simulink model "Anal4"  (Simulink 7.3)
settings: Solver=ode45  StartTime=0.0  StopTime=10.0  RelTol=1e-3
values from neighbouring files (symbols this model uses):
  d2r = 1/r2d    (= 0.0174532925199)    [run.m]
  Kp3 = [0.3042  3.4539  0.5105  0.0711 -0.2670]    [run.m]
  Thr = [470000, 470000, 470000, 0.245e7, 0.245e7]'    [run.m]
undefined symbols (not defined in the file or in its folder): Ap, Bp, Cp, Cza, Dp, Mass, Qbar, Sref, TVC

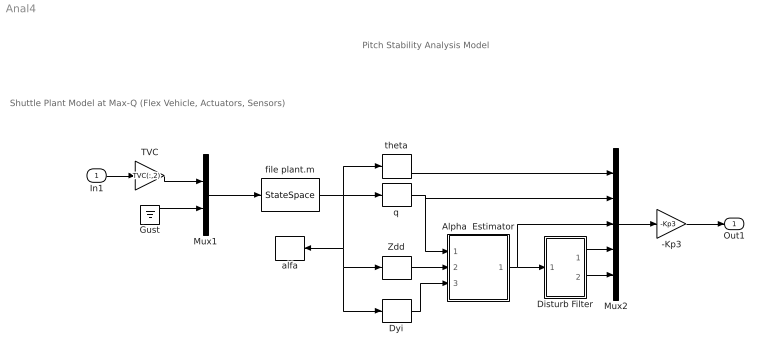
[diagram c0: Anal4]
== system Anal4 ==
  note: Shuttle Plant Model at Max-Q (Flex Vehicle, Actuators, Sensors)
  note: Pitch Stability Analysis Model
  In1 : Inport  OutDataType=sfix(16)  OutScaling=2^0
  -Kp3 : Gain  Gain=-Kp3  Multiplication=Matrix(K*u)  ParameterDataType=sfix(16)  ParameterScaling=2^0  OutDataType=sfix(16)  OutScaling=2^0
  Alpha  Estimator : Subsystem
  Disturb Filter : Subsystem
  Dyi : Selector  InputPortWidth=30  IndexOptions=Index vector (dialog)  Indices=[21:25]  OutputSizes=1
  Gust : Ground
  Mux1 : Mux  Inputs=[10,1]
  Mux2 : Mux  Inputs=5
  TVC : Gain  Gain=TVC(:,2)  Multiplication=Matrix(K*u)  ParameterDataType=sfix(16)  ParameterScaling=2^0  OutDataType=sfix(16)  OutScaling=2^0
  Zdd : Selector  InputPortWidth=30  IndexOptions=Index vector (dialog)  Indices=[8]  OutputSizes=1
  alfa : Selector  InputPortWidth=30  IndexOptions=Index vector (dialog)  Indices=[9]  OutputSizes=1
  file plant.m : StateSpace  A=Ap  B=Bp  C=Cp  D=Dp
  q : Selector  InputPortWidth=30  IndexOptions=Index vector (dialog)  Indices=[5]  OutputSizes=1
  theta : Selector  InputPortWidth=30  IndexOptions=Index vector (dialog)  Indices=[2]  OutputSizes=1
  Out1 : Outport  OutDataType=sfix(16)  OutScaling=2^0
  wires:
  Mux2/1 -> -Kp3/1
  Disturb Filter/1(x1) -> Mux2/4
  Disturb Filter/2(x2) -> Mux2/5
  theta/1 -> Mux2/1
  q/1 -> Mux2/2, Alpha  Estimator/1(q)
  file plant.m/1 -> theta/1, q/1, alfa/1, Zdd/1, Dyi/1
  Mux1/1 -> file plant.m/1
  TVC/1 -> Mux1/1
  In1/1 -> TVC/1
  -Kp3/1 -> Out1/1
  Alpha  Estimator/1(alphat) -> Disturb Filter/1(alfa), Mux2/3
  Zdd/1 -> Alpha  Estimator/2(Zdd)
  Dyi/1 -> Alpha  Estimator/3(delta)
  Gust/1 -> Mux1/2

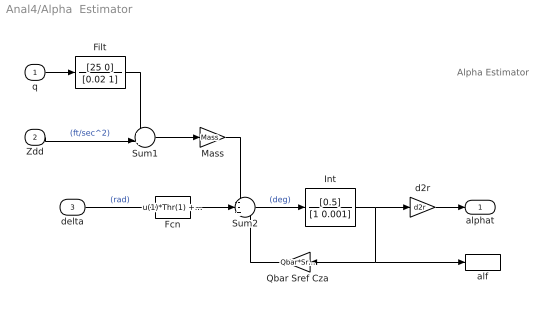
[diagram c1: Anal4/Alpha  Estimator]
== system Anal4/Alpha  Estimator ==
  note: Alpha Estimator
  q : Inport  OutDataType=sfix(16)  OutScaling=2^0
  Zdd : Inport  Port=2  OutDataType=sfix(16)  OutScaling=2^0
  delta : Inport  Port=3  OutDataType=sfix(16)  OutScaling=2^0
  Fcn : Fcn  Expr=u(1)*Thr(1) +u(2)*Thr(2) +u(3)*Thr(3) +u(4)*Thr(4) +u(5)*Thr(5)
  Filt : TransferFcn  Numerator=[25 0]  Denominator=[0.02 1]
  Int : TransferFcn  Numerator=[0.5]  Denominator=[1 0.001]
  Mass : Gain  Gain=Mass  ParameterDataType=sfix(16)  ParameterScaling=2^0  OutDataType=sfix(16)  OutScaling=2^0
  Qbar Sref Cza : Gain  Gain=Qbar*Sref*Cza  ParameterDataType=sfix(16)  ParameterScaling=2^0  OutDataType=sfix(16)  OutScaling=2^0
  Sum1 : Sum  Inputs=++|  OutDataType=sfix(16)  OutScaling=2^0
  Sum2 : Sum  Inputs=--+  OutDataType=sfix(16)  OutScaling=2^0
  alf : ToWorkspace  VariableName=alphat  SampleTime=-1  SaveFormat=Array
  d2r : Gain  Gain=d2r  ParameterDataType=sfix(16)  ParameterScaling=2^0  OutDataType=sfix(16)  OutScaling=2^0
  alphat : Outport  OutDataType=sfix(16)  OutScaling=2^0
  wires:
  Fcn/1 -> Sum2/2
  Filt/1 -> Sum1/1
  Sum1/1 -> Mass/1
  Zdd/1 -> Sum1/2  "(ft/sec^2)"
  q/1 -> Filt/1
  Sum2/1 -> Int/1  "(deg)"
  Qbar Sref Cza/1 -> Sum2/3
  delta/1 -> Fcn/1  "(rad)"
  Mass/1 -> Sum2/1
  d2r/1 -> alphat/1
  Int/1 -> d2r/1, Qbar Sref Cza/1, alf/1

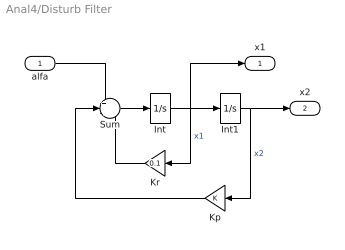
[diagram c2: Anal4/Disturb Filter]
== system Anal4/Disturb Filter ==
  alfa : Inport  OutDataType=sfix(16)  OutScaling=2^0
  Int : Integrator
  Int1 : Integrator
  Kp : Gain  ParameterDataType=sfix(16)  ParameterScaling=2^0  OutDataType=sfix(16)  OutScaling=2^0
  Kr : Gain  Gain=0.1  ParameterDataType=sfix(16)  ParameterScaling=2^0  OutDataType=sfix(16)  OutScaling=2^0
  Sum : Sum  Inputs=+--  OutDataType=sfix(16)  OutScaling=2^0
  x1 : Outport  OutDataType=sfix(16)  OutScaling=2^0
  x2 : Outport  Port=2  OutDataType=sfix(16)  OutScaling=2^0
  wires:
  Int/1 -> Int1/1, Kr/1, x1/1  "x1"
  Sum/1 -> Int/1
  Int1/1 -> Kp/1, x2/1  "x2"
  Kr/1 -> Sum/3
  Kp/1 -> Sum/2
  alfa/1 -> Sum/1
